|//////////////////////////////////////////////////////////////////////////////
|//////////////////////////////////////////////////////////////////////////////
|   @@@@@@@   @@@@@@@   @@@@@@@   @@@@@@@   @@@@@@@   @@@@@@   @@
|   @@@@@@@@@   @@@@@@@@@   @@@@@@@@@   @@@@@@@@@   @@@@@@@@@ @@@@@@@@  @
|   @@@   @@@ @@@   @@@ @@@   @@@   @@@ @@@   @@@@   @@@  @
|   @@   @@ @@   @@ @@@@@@@@@@@ @@@@@@@@@@@ @@   @@   @@ @@
|   @@@   @@@ @@   @@   @@@ @@@   @@   @@   @@ @@
|   @@@@@@@@@  @@   @@  @@@@@@@@@   @@@@@@@@@  @@   @@   @@ @@
|   @@@@@@@   @@   @@   @@@@@@@   @@@@@@@   @@   @@   @@ @@
|   IBIS Model of MC74VHC1G125
|   Single Non-Inverting Buffer, 3-State
|   Package Type:  SC-88A/SC-70-5, CASE 419A-02 (DF)
|   SC-74A, CASE 318BQ (DBV)
|   SOT-953, CASE 527AE (P5)
|   The model is covering the following Vccs:
|   2.0V, 2.5V, 3.3V, 5.0V
|//////////////////////////////////////////////////////////////////////////////
|//////////////////////////////////////////////////////////////////////////////
[IBIS Ver]   3.2
|   7.2 compatible
|//////////////////////////////////////////////////////////////////////////////
[Comment Char] |_char
|//////////////////////////////////////////////////////////////////////////////
[File Name]   74vhc1g125_va_r0.ibs
|//////////////////////////////////////////////////////////////////////////////
[File Rev]   0.0
|   0.0 - February 27, 2024 - File created
|//////////////////////////////////////////////////////////////////////////////
[Date]   Feb 27, 2024
|//////////////////////////////////////////////////////////////////////////////
[Source]   From lab measurements and simulations at onsemi
|//////////////////////////////////////////////////////////////////////////////
[Notes]
   - The currents greater than +/- 100 mA are extrapolated
|//////////////////////////////////////////////////////////////////////////////
[Disclaimer]
   - onsemi Corporation hereby grants
   the user of this IBIS model a license to use this model
   under the following terms. This license is nonexclusive
   and nontransferable. Before using this IBIS model.
   After reading the terms and conditions of this license,
   the user either must accept these terms,
   or the IBIS model should be returned to onsemi within 30 days.
   - The user is hereby granted a license to use the IBIS model.
   This shall not be construed as a right to sell,
   or otherwise profit either by leasing or renting this software.
   - The user may modify the IBIS model to suit his specific
   applications but rights to derivative works and such
   modifications shall belong to onsemi.
   - This IBIS model is provided on an "as is" basis.
   onsemi makes absolutely no warranty with respect
   to the information contained herein.
   By use of this IBIS model, the user assumes full risk as to the
   quality and suitablility of the model to his particular use,
   and by using this model assumes the entire risk.
   Under all circumstances the user shall not hold
   onsemi liable in any way for the results obtained.
   onsemi reserves the right to make to improve
   the model for reliability, function, or design.
   onsemi does not convey any license under patent
   rights or any other intellectual property rights,
   including those of third parties.
   - onsemi is not obligated to provide maintenance
   or support for the licensed IBIS model.
   - Cont onsemi at ATTN:LOGIC APPLICATIONS/IBIS MODEL.
   5701 N Pima Rd, Scottsdale, AZ 85250
|//////////////////////////////////////////////////////////////////////////////
[Copyright]   (c) 2024 onsemi Corp.
|//////////////////////////////////////////////////////////////////////////////
|//////////////////////////////////////////////////////////////////////////////
|[Component]   M74VHC1G125DTT1G
||//////////////////////////////////////////////////////////////////////////////
|[Manufacturer]  onsemi
||   Data Sheet:   MC74VHC1G125/D, Rev. 23,  Aug, 2023
||//////////////////////////////////////////////////////////////////////////////
|[Package]
|| TSOP-5/SOT-23-5
||   DT SUFFIX
||   CASE 483
|| variable   typ   min   max
|R_pkg   0.02532   0.0216   0.0295
|L_pkg   1.52928nH   1.3125nH   1.9067nH
|C_pkg   0.15688pF   0.1108pF   0.2403pF
||//////////////////////////////////////////////////////////////////////////////
|[Pin]   signal_name   model_name   R_pin   L_pin   C_pin
|1   OE   In   0.0216   1.5112nH   0.1443pF
|2   A   In   0.0237   1.3125nH   0.1382pF
|3   GND   GND   0.0295   1.9067nH   0.2403pF
|4   Y   Out   0.0266   1.5415nH   0.1508pF
|5   VCC   POWER   0.0252   1.3745nH   0.1108pF
||//////////////////////////////////////////////////////////////////////////////
||//////////////////////////////////////////////////////////////////////////////
[Component]   M74VHC1G125DFT1G
|//////////////////////////////////////////////////////////////////////////////
[Manufacturer]  onsemi
|   Data Sheet:   MC74VHC1G125/D, Rev. 23,  Aug, 2023
|//////////////////////////////////////////////////////////////////////////////
[Package]
| SC-88A / SC-70-5
|   DF SUFFIX
|   CASE 419A-02
| variable   typ   min   max
R_pkg   0.0201   0.0170   0.0250
L_pkg   0.9982nH   0.8810nH   1.0690nH
C_pkg   0.1466pF   0.1187pF   0.2051pF
|//////////////////////////////////////////////////////////////////////////////
[Pin]   signal_name   model_name   R_pin   L_pin   C_pin
1   OE   In   0.0191   1.0690nH   0.1625pF
2   A   In   0.0187   0.8810nH   0.1217pF
3   GND   GND   0.0170   1.0315nH   0.2051pF
4   Y   Out   0.0207   0.9600nH   0.1249pF
5   VCC   POWER   0.0250   1.0497nH   0.1187pF
|//////////////////////////////////////////////////////////////////////////////
|//////////////////////////////////////////////////////////////////////////////
[Component]   M74VHC1G125DFT2G
|//////////////////////////////////////////////////////////////////////////////
[Manufacturer]  onsemi
|   Data Sheet:   MC74VHC1G125/D, Rev. 23,  Aug, 2023
|//////////////////////////////////////////////////////////////////////////////
[Package]
R_pkg   0.0201   0.0170   0.0250
L_pkg   0.9982nH   0.8810nH   1.0690nH
C_pkg   0.1466pF   0.1187pF   0.2051pF
|//////////////////////////////////////////////////////////////////////////////
[Pin]   signal_name   model_name   R_pin   L_pin   C_pin
1   OE   In   0.0191   1.0690nH   0.1625pF
2   A   In   0.0187   0.8810nH   0.1217pF
3   GND   GND   0.0170   1.0315nH   0.2051pF
4   Y   Out   0.0207   0.9600nH   0.1249pF
5   VCC   POWER   0.0250   1.0497nH   0.1187pF
|//////////////////////////////////////////////////////////////////////////////
|//////////////////////////////////////////////////////////////////////////////
[Component]   M74VHC1G125DFT1G-Q
|//////////////////////////////////////////////////////////////////////////////
[Manufacturer]  onsemi
|   Data Sheet:   MC74VHC1G125/D, Rev. 23,  Aug, 2023
|//////////////////////////////////////////////////////////////////////////////
[Package]
R_pkg   0.0201   0.0170   0.0250
L_pkg   0.9982nH   0.8810nH   1.0690nH
C_pkg   0.1466pF   0.1187pF   0.2051pF
|//////////////////////////////////////////////////////////////////////////////
[Pin]   signal_name   model_name   R_pin   L_pin   C_pin
1   OE   In   0.0191   1.0690nH   0.1625pF
2   A   In   0.0187   0.8810nH   0.1217pF
3   GND   GND   0.0170   1.0315nH   0.2051pF
4   Y   Out   0.0207   0.9600nH   0.1249pF
5   VCC   POWER   0.0250   1.0497nH   0.1187pF
|//////////////////////////////////////////////////////////////////////////////
|//////////////////////////////////////////////////////////////////////////////
[Component]   M74VHC1G125DFT2G-Q
|//////////////////////////////////////////////////////////////////////////////
[Manufacturer]  onsemi
|   Data Sheet:   MC74VHC1G125/D, Rev. 23,  Aug, 2023
|//////////////////////////////////////////////////////////////////////////////
[Package]
R_pkg   0.0201   0.0170   0.0250
L_pkg   0.9982nH   0.8810nH   1.0690nH
C_pkg   0.1466pF   0.1187pF   0.2051pF
|//////////////////////////////////////////////////////////////////////////////
[Pin]   signal_name   model_name   R_pin   L_pin   C_pin
1   OE   In   0.0191   1.0690nH   0.1625pF
2   A   In   0.0187   0.8810nH   0.1217pF
3   GND   GND   0.0170   1.0315nH   0.2051pF
4   Y   Out   0.0207   0.9600nH   0.1249pF
5   VCC   POWER   0.0250   1.0497nH   0.1187pF
|//////////////////////////////////////////////////////////////////////////////
|//////////////////////////////////////////////////////////////////////////////
[Component]   MC74VHC1G125DBVT1G
|//////////////////////////////////////////////////////////////////////////////
[Manufacturer]  onsemi
|   Data Sheet:   MC74VHC1G125/D, Rev. 23,  Aug, 2023
|//////////////////////////////////////////////////////////////////////////////
[Package]
|  SC-74A
| DBV SUFFIX
| CASE 318BQ
| variable   typ   min   max
R_pkg   0.0710   0.0522   0.0935
L_pkg   1.2331nH   1.0634nH   1.4484nH
C_pkg   0.1280pF   0.1167pF   0.1367pF
|//////////////////////////////////////////////////////////////////////////////
[Pin]   signal_name   model_name   R_pin   L_pin   C_pin
1   OE   In   0.0522   1.0634nH   0.1235pF
2   A   In   0.0588   1.1995nH   0.1367pF
3   GND   GND   0.0828   1.3327nH   0.1351pF
4   Y   Out   0.0935   1.4484nH   0.1279pF
5   VCC   POWER   0.0679   1.1215nH   0.1167pF
|//////////////////////////////////////////////////////////////////////////////
|//////////////////////////////////////////////////////////////////////////////
[Component]   MC74VHC1G125P5T5G
|//////////////////////////////////////////////////////////////////////////////
[Manufacturer]  onsemi
|   Data Sheet:   MC74VHC1G125/D, Rev. 23,  Aug, 2023
|//////////////////////////////////////////////////////////////////////////////
[Package]
|  SOT-953
| P5  SUFFIX
| CASE 527AE
| variable   typ   min   max
R_pkg   0.0786   0.0731   0.0817
L_pkg   1.1377nH   1.0330nH   1.1757nH
C_pkg   0.0487pF   0.0295pF   0.0642pF
|//////////////////////////////////////////////////////////////////////////////
[Pin]   signal_name   model_name   R_pin   L_pin   C_pin
1   A   In   0.0817   1.1757nH   0.0433pF
2   GND   GND   0.0731   1.0330nH   0.0295pF
3   OE   In   0.0805   1.1531nH   0.0500pF
4   Y   Out   0.0789   1.1637nH   0.0642pF
5   VCC   POWER   0.0787   1.1630nH   0.0567pF
|//////////////////////////////////////////////////////////////////////////////
|//////////////////////////////////////////////////////////////////////////////
[Model Selector]   In
In_20   Vcc = 2.00
In_25   Vcc = 2.50
In_33   Vcc = 3.30
In_50   Vcc = 5.00
|//////////////////////////////////////////////////////////////////////////////
[Model Selector]   Out
Out_20   Vcc = 2.00
Out_25   Vcc = 2.50
Out_33   Vcc = 3.30
Out_50   Vcc = 5.00
| Models and submodels in the file (8): In_20 (Input), Out_20 (3-state), In_25 (Input), Out_25 (3-state), In_33 (Input), Out_33 (3-state), In_50 (Input), Out_50 (3-state)
